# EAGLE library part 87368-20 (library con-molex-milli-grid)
RECEPTACAL
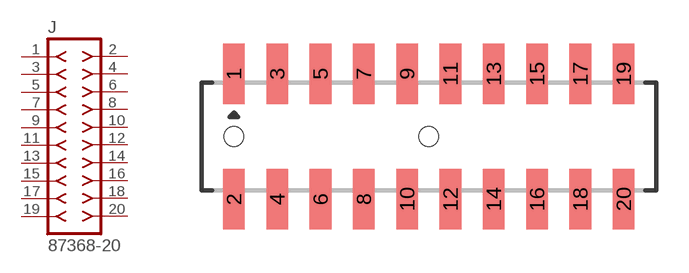
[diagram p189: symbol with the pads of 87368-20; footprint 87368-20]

Designator prefix J

## 87368-20  [87368-20]
1  1  pas
2  2  pas
3  3  pas
4  4  pas
5  5  pas
6  6  pas
7  7  pas
8  8  pas
9  9  pas
10  10  pas
11  11  pas
12  12  pas
13  13  pas
14  14  pas
15  15  pas
16  16  pas
17  17  pas
18  18  pas
19  19  pas
20  20  pas

## Footprint 87368-20 (pad centres in mm)
RECEPTACAL SMD Dual Row, Side Entry
smd 1 x 2.8: 1 -9,2.9; 2 -9,-2.9; 3 -7,2.9; 4 -7,-2.9; 5 -5,2.9; 6 -5,-2.9; 7 -3,2.9; 8 -3,-2.9; 9 -1,2.9; 10 -1,-2.9; 11 1,2.9; 12 1,-2.9; 13 3,2.9; 14 3,-2.9; 15 5,2.9; 16 5,-2.9; 17 7,2.9; 18 7,-2.9; 19 9,2.9; 20 9,-2.9
hole 0.914 at -9,0
hole 0.914 at 0,0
